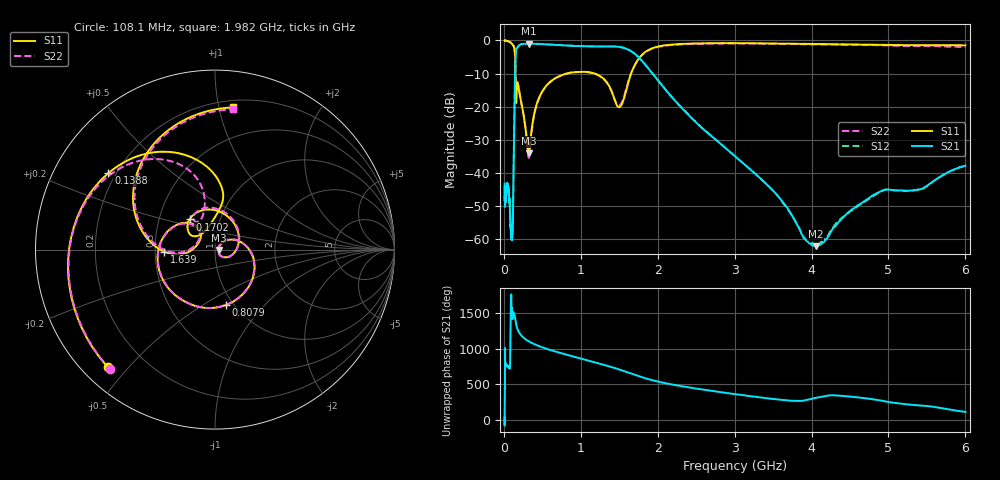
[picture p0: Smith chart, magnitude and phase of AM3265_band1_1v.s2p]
!Agilent Technologies,E8364B,MY43040894,A.07.50.67
!Agilent E8364B: A.07.50.67
!Date: Friday, May 09, 2025 07:13:37
!Correction: S11(Full 2 Port(1,2))
!S21(Full 2 Port(1,2))
!S12(Full 2 Port(1,2))
!S22(Full 2 Port(1,2))
!S2P File: Measurements: S11, S21, S12, S22:Log Frequency Sweep
# Hz S  dB  R 50
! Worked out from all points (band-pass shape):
!   3201 points, 10 MHz to 6 GHz, reference 50 ohm
!   highest |S21| = -0.95 dB at 329.9 MHz (marker M1); lowest = -62.1 dB at 4.055 GHz (marker M2)
!   |S21| within 3 dB of the highest: 155.5 MHz to 1.698 GHz (1.543 GHz wide, 166 % of centre)
!   lowest |S11| = -34.0 dB at 320.8 MHz (marker M3), VSWR 1.04, Z = 52 - j0.196 ohm
!   |S11| at or under -10 dB: 149.6 MHz to 814.5 MHz (664.9 MHz wide, 138 % of centre); 1.185 GHz to 1.653 GHz (468.7 MHz wide, 33 % of centre)
!   |S22| runs from -35.4 to 0.0 dB; largest |S21 - S12| = 0.013
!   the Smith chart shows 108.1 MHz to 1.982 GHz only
!   S11 on the Smith chart (normalised r, x): 108.1 MHz: 0.07, -0.44; 138.8 MHz: 0.17, +0.31; 170.2 MHz: 0.71, +0.25; 807.9 MHz: 0.92, -0.63; 1.639 GHz: 0.56, -0.01; 1.982 GHz: 0.25, +1.10
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1e7  -0.03 -10.2  -43.16 30.8  -44.01 -126.8  -0.06 -10.0
2.908064e7  -0.07 -29.3  -44.93 61.1  -44.71 63.2  -0.07 -29.3
8.439949e7  -0.53 -94.1  -53.93 -9.0  -54.38 138.0  -0.56 -93.9
1.081417e8  -1.05 -132.3  -59.59 46.6  -57.47 98.1  -1.05 -131.1
1.3884e8  -2.72 144.4  -19.33 34.8  -19.26 34.9  -2.60 150.9
1.702426e8  -13.15 130.2  -2.33 -141.7  -2.29 -141.7  -12.66 117.0
2.44949e8  -20.93 -25.2  -1.06 86.6  -1.03 86.5  -20.93 -25.3
3.208329e8  -34.00 -5.4  -0.95 26.0  -0.92 25.9  -35.29 -11.6
3.299387e8  -33.37 14.2  -0.95 20.3  -0.92 20.3  -35.02 12.5
7.123273e8  -10.88 -52.9  -1.38 -132.3  -1.35 -132.3  -10.88 -53.3
8.079314e8  -10.04 -79.0  -1.51 -161.6  -1.48 -161.6  -10.04 -79.6
1.197855e9  -10.11 177.3  -1.80 84.9  -1.77 84.9  -10.19 176.5
1.442595e9  -18.06 129.7  -1.81 8.6  -1.77 8.6  -17.88 132.2
1.639485e9  -10.93 -177.8  -3.04 -63.4  -3.01 -63.3  -10.80 179.7
1.982366e9  -1.95 82.7  -11.45 -176.3  -11.43 -176.2  -2.07 82.8
2.067357e9  -1.55 62.6  -13.89 163.2  -13.87 163.2  -1.67 63.0
2.455151e9  -0.91 -11.2  -23.72 87.6  -23.69 87.6  -1.05 -10.5
2.96862e9  -0.79 -90.2  -34.21 6.8  -34.16 7.1  -0.90 -90.3
3.518433e9  -0.90 -166.6  -45.78 -68.2  -45.74 -69.5  -1.00 -168.4
4.054987e9  -1.07 123.1  -62.06 -50.1  -61.39 -47.5  -1.17 120.7
5.002045e9  -1.35 4.2  -44.99 -108.8  -45.03 -108.5  -1.53 4.7
6e9  -1.45 -115.3  -37.79 112.3  -37.76 111.9  -1.96 -111.0
